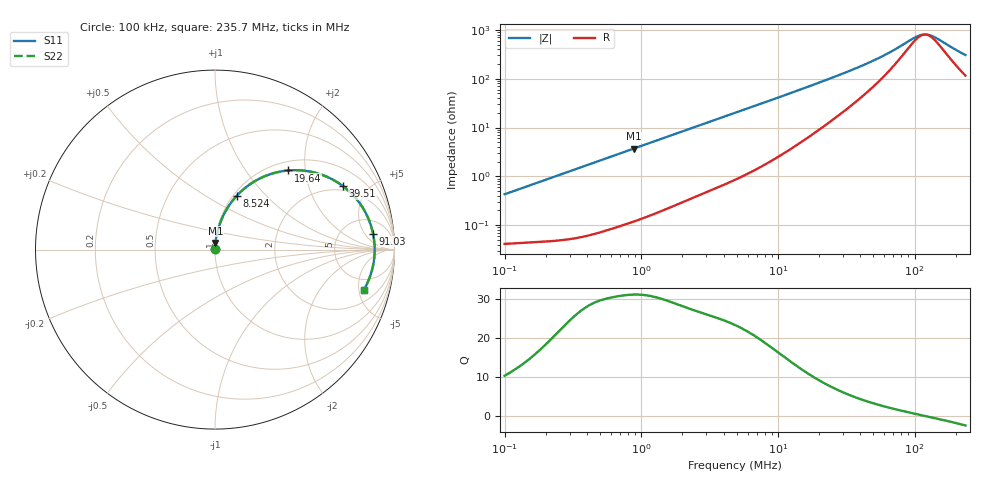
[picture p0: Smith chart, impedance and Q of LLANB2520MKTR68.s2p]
! LLANB2520MKTR68  S-PARAMETER MODEL  ( General Type )
! Model Generated by TAIYO YUDEN Corporation (http://www.ty-top.com)
! Version 2.0
! TAIYO YUDEN Control No. 20210629
! Copyright(c) 2012 TAIYO YUDEN CO.,LTD. All Rights Reserved.
! Product Description (link to TY-COMPAS)
! https://ds.yuden.co.jp/TYCOMPAS/or/detail?pn=LLANB2520MKTR68M&u=M
! Products Name : Inductors
! Characteristics :
!  Inductance : 0.68 uH , SRF(min) : -Hz , DC Resistance(max) : 0.048 Ohm
!  Rated Current : Saturation :3200 mA , Temp Rise : 3200 mA (40 degC)
!  Case Size : 2.5 x 2.0 / 0.098 x 0.079 [mm/inch] , Thickness : 1.2 / 0.047 [mm/inch]
!  (Conditions: Temperature = 25 degC , DC Bias Current/Voltage = 0A / 0V)
! External Node Assignments :
!  1  o---GGG---o  2
! GND o---------o GND
! Frequency Range : 0.1MHz  -  235.669543MHz  [ 402 STEP ]
# MHz S RI R 50
! Freq[MHz].  S11 Real  S11 Imag  S21 Real  S21 Imag  S12 Real  S12 Imag  S22 Real  S22 Imag
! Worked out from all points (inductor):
!   401 points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, 100 kHz to 235.7 MHz, reference 50 ohm
!   read as one part in series: L = 677 nH near 104 kHz
!   highest Q = 31.3 at 879.5 kHz (marker M1), where L = 668 nH
!   self-resonance near 119.4 MHz
!   S11 on the Smith chart (normalised r, x): 100 kHz: 1.00, +0.01; 8.524 MHz: 1.04, +0.69; 19.64 MHz: 1.17, +1.62; 39.51 MHz: 1.77, +3.42; 91.03 MHz: 10, +8; 235.7 MHz: 3.31, -5.66
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0.1  0.00043 0.00426  0.9996 -0.00426  0.9996 -0.00426  0.00043 0.00426
0.367165  0.000811 0.0155  0.9992 -0.0155  0.9992 -0.0155  0.000811 0.0155
0.879518  0.00254 0.0368  0.9975 -0.0368  0.9975 -0.0368  0.00254 0.0368
1.348099  0.00499 0.0559  0.995 -0.0559  0.995 -0.0559  0.00499 0.0559
2.711621  0.0164 0.1095  0.9836 -0.1095  0.9836 -0.1095  0.0164 0.1095
4.854581  0.0454 0.1878  0.9546 -0.1878  0.9546 -0.1878  0.0454 0.1878
8.524006  0.1209 0.2997  0.8791 -0.2997  0.8791 -0.2997  0.1209 0.2997
12.32617  0.2191 0.3795  0.7809 -0.3795  0.7809 -0.3795  0.2191 0.3795
17.8243  0.3641 0.4348  0.6359 -0.4348  0.6359 -0.4348  0.3641 0.4348
19.64112  0.4083 0.4409  0.5917 -0.4409  0.5917 -0.4409  0.4083 0.4409
27.32054  0.563 0.4271  0.437 -0.4271  0.437 -0.4271  0.563 0.4271
39.50697  0.7143 0.3527  0.2857 -0.3527  0.2857 -0.3527  0.7143 0.3527
51.84469  0.7954 0.2729  0.2046 -0.2729  0.2046 -0.2729  0.7954 0.2729
65.44454  0.843 0.1976  0.157 -0.1976  0.157 -0.1976  0.843 0.1976
91.03246  0.8806 0.0889  0.1194 -0.0889  0.1194 -0.0889  0.8806 0.0889
102.2777  0.8867 0.0507  0.1133 -0.0507  0.1133 -0.0507  0.8867 0.0507
110.536  0.8889 0.0253  0.1111 -0.0253  0.1111 -0.0253  0.8889 0.0253
119.4612  0.8897 -0.000121  0.1103 0.000121  0.1103 0.000121  0.8897 -0.000121
126.6249  0.8893 -0.0192  0.1107 0.0192  0.1107 0.0192  0.8893 -0.0192
142.2669  0.886 -0.0573  0.114 0.0573  0.114 0.0573  0.886 -0.0573
197.8913  0.8576 -0.166  0.1424 0.166  0.1424 0.166  0.8576 -0.166
235.6695  0.8295 -0.2236  0.1705 0.2236  0.1705 0.2236  0.8295 -0.2236
